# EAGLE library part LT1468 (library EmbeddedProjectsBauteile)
LINEAR TECHNOLOGY LT1468CS8#PBF - OP-VERST,90MHZ,22V/US,8SOIC
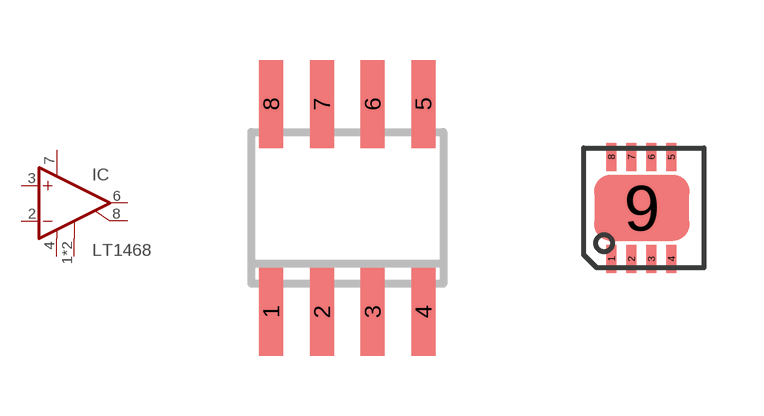
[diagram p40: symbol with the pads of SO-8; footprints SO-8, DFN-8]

Designator prefix IC

## LT1468CS8  [SO-8]
1  NC  nc
2  -IN  in
3  +IN  in
4  V-  pwr
5  NC  nc
6  OUT  out
7  V+  pwr
8  SHDN  pas

## LT1468ACCD (EP: 401439)  [DFN-8]
1  NC  nc
2  -IN  in
3  +IN  in
4  V-  pwr
5  NC  nc
6  OUT  out
7  V+  pwr
8  SHDN  pas
9  V-  pwr

## Footprint SO-8 (pad centres in mm)
smd 0.6 x 2.2: 1 -1.905,-2.6; 2 -0.635,-2.6; 3 0.635,-2.6; 4 1.905,-2.6; 5 1.905,2.6; 6 0.635,2.6; 7 -0.635,2.6; 8 -1.905,2.6

## Footprint DFN-8 (pad centres in mm)
smd 0.25 x 0.7: 1 0.688,0.223; 2 1.188,0.223; 3 1.688,0.223; 4 2.188,0.223; 5 2.188,2.777; 6 1.688,2.777; 7 1.188,2.777; 8 0.688,2.777
smd 2.38 x 1.65: 9 1.45,1.5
